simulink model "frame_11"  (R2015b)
settings: Solver=FixedStepDiscrete  StartTime=0.0  StopTime=20  RelTol=1e-3
undefined symbols (not defined in the file or in its folder): fir1
libraries: simulink x1, dspstat3 x1

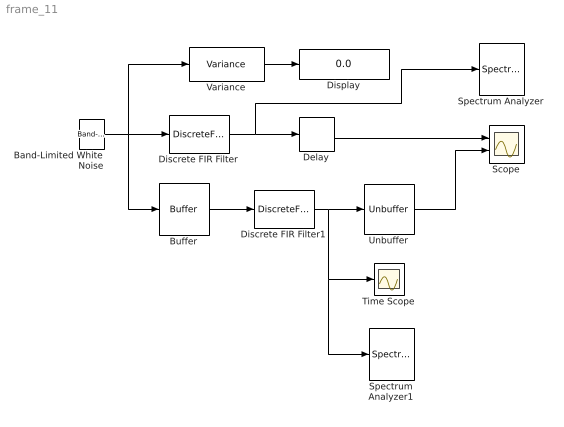
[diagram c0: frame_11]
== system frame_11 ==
  Band-Limited White Noise : simulink/Sources/Band-Limited White Noise  Cov=1/1000  Ts=1/1000  seed=[23341]
  Buffer : Buffer  N=512*4  TreatMby1Signals=One channel  OutputFrames=off
  Delay : Delay  DelayLength=2*2048
  Discrete FIR Filter : DiscreteFir  Coefficients=fir1(64, 0.5);
  Discrete FIR Filter1 : DiscreteFir  Coefficients=fir1(64, 0.5);  InputProcessing=Columns as channels (frame based)
  Display : Display
  Scope : Scope  NumInputPorts=2
  Spectrum Analyzer : SpectrumAnalyzer
  Spectrum Analyzer1 : SpectrumAnalyzer
  Time Scope : Scope
  Unbuffer : Unbuffer  SampleBasedProcessing=Same as frame based
  Variance : dspstat3/Variance  run=on  reset_popup=None  directionMode=Each column  dimension=1  roiEnable=off  roiType=Rectangles  roiPortion=Entire ROI  roiOutput=Individual statistics for each ROI  roiFlag=off  roundingMode=Floor  overflowMode=off
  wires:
  Band-Limited White Noise/1 -> Variance/1, Discrete FIR Filter/1, Buffer/1
  Discrete FIR Filter1/1 -> Spectrum Analyzer1/1, Time Scope/1, Unbuffer/1
  Unbuffer/1 -> Scope/2
  Delay/1 -> Scope/1
  Variance/1 -> Display/1
  Buffer/1 -> Discrete FIR Filter1/1
  Discrete FIR Filter/1 -> Delay/1, Spectrum Analyzer/1
